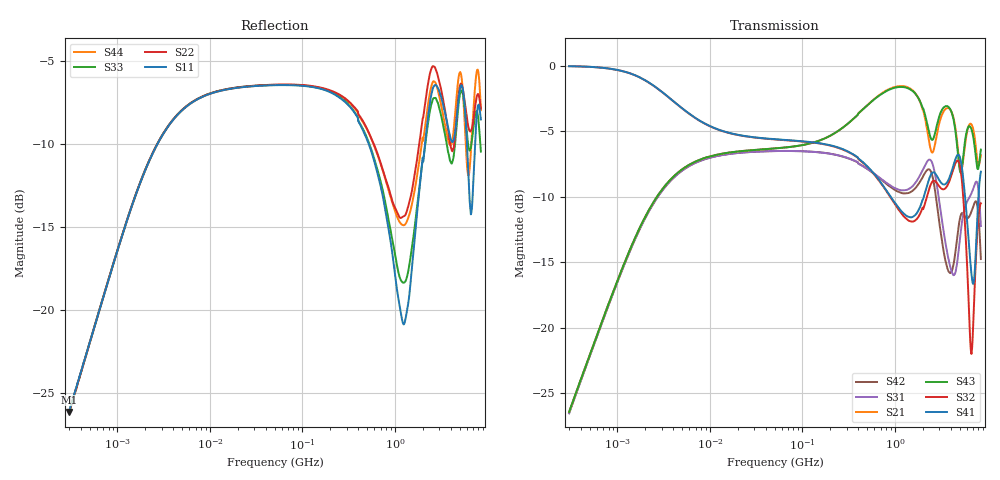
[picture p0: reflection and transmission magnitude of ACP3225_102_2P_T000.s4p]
! S-Parameter Data Generated by TDK Corporation
! Copyright(C) 2020 TDK Corporation.
! All Rights Reserved.
! TDK P/N: ACP3225-102-2P-T000 (Common Mode Filter)
! Property: |Zc|=1000ohm at 100MHz
! Size(LxWxT): 3.2x2.5x1.9mm
! Model Type: s4p (Touchstone File Format Version 1.0)
! Frequency: DC=Yes Start=0.3MHz Stop=8500MHz 802points Log-sweep
! Model Generated on Aug. 18, 2020
! Port Assignments:
!  1 ---@@@--- 4
!  2 ---@@@--- 3
! Applicable Conditions:
!  Temperature = 25 degC
!  DC Bias Current = 0 A
!  Small Signal Operation
! Terms and conditions regarding TDK Simulation Models
! (1)This simulation model is being provided solely for informational purposes. Please refer to the specifications of the products in terms of detailed characteristics of such products.
! (2)In no event shall TDK Corporation of any of its subsidiaries be liable for any loss or damage arising, directly or indirectly,
!  From any information contained in this simulation model, including, but not limited to loss or damages arising from any inaccuracies, omissions or errors in connection with such information.
! (3)Any and all copyrights on this simulation model are owned by TDK Corporation.
!  Duplication or redistribution of this simulation model without prior written permission from TDK Corporation is prohibited.
! (4)This simulation model is subject to any modification or change without any prior notice.
! (5)Neither TDK Corporation nor any of its subsidiaries shall make any warranty, express or implied,
!  Including but not limited to the correctness, implied warranties of merchantability and fitness for a particular purpose with respect to this simulation models.
! (6)The use of this simulation model shall be deemed to have consented to the terms and conditions hereof.
# Hz S MA R 50
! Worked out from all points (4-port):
!   801 points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, 300 kHz to 8.5 GHz, reference 50 ohm
!   strongest paths, dB at 300 kHz, 3.892 MHz, 50.5 MHz, 655.2 MHz, 8.5 GHz:
!     S41: 0.0, -2.6, -5.6, -8.6, -8.1
!     S32: -0.1, -2.6, -5.6, -8.7, -10.5
!     S43: -26.4, -8.6, -6.3, -2.4, -6.4
!     S21: -26.4, -8.6, -6.3, -2.3, -6.9
!     S31: -26.5, -8.7, -6.5, -8.5, -12.2
!     S42: -26.5, -8.7, -6.5, -8.5, -14.8
!   lowest |S11| = -26.1 dB at 300 kHz (marker M1), VSWR 1.10, Z = 50.2 + j4.94 ohm
!   |S11| at or under -10 dB: start of sweep to 2.704 MHz; 521 MHz to 2.114 GHz (1.593 GHz wide, 121 % of centre); 6.015 GHz to 7.348 GHz (1.333 GHz wide, 20 % of centre)
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300000  0.0493 84.9  0.04772 83.8  0.04725 -96.3  0.9957 -2.8
        0.04763 83.8  0.04881 84.0  0.9948 -2.7  0.0472 -96.3
        0.04712 -96.3  0.9942 -2.7  0.04936 84.4  0.04773 83.6
        0.9945 -2.7  0.0472 -96.3  0.04772 83.7  0.04916 84.6
8938596  0.4428 18.0  0.445 19.5  0.4401 -162.4  0.5992 -14.9
         0.445 19.5  0.4439 18.2  0.5982 -15.0  0.4401 -162.2
         0.4401 -162.4  0.5981 -15.0  0.4438 18.0  0.4451 19.5
         0.5992 -14.9  0.44 -162.2  0.4451 19.5  0.4428 18.2
1.010223e9  0.1257 -51.6  0.8295 -9.6  0.3402 75.5  0.2984 -91.3
            0.8294 -9.6  0.2024 -30.1  0.2941 -93.1  0.3344 89.8
            0.3401 75.4  0.2942 -93.1  0.1454 -47.8  0.8237 -9.6
            0.298 -91.3  0.3342 89.9  0.8238 -9.6  0.1972 -32.3
2.784768e9  0.4754 -73.5  0.526 -30.4  0.3665 -52.3  0.3842 108.6
            0.5252 -30.3  0.5265 -74.5  0.362 96.4  0.313 -50.7
            0.3653 -52.2  0.3592 96.2  0.4328 -81.3  0.5737 -33.9
            0.3833 108.7  0.3127 -50.6  0.5741 -33.9  0.4787 -73.2
5.489348e9  0.452 -99.1  0.4371 -58.1  0.2711 58.6  0.3666 -63.1
            0.4404 -57.4  0.4544 -94.1  0.3129 -84.3  0.2728 59.6
            0.2716 59.8  0.3125 -82.3  0.4391 -103.2  0.4541 -61.2
            0.3683 -63.6  0.2714 59.7  0.4525 -60.6  0.435 -96.7
6.718408e9  0.1967 -77.5  0.5953 -82.3  0.3202 -18.8  0.1609 -151.1
            0.5966 -83.0  0.3493 -87.1  0.08083 138.7  0.2786 -8.7
            0.3251 -18.1  0.07934 145.6  0.3169 -89.9  0.569 -90.9
            0.1601 -149.9  0.2769 -8.1  0.5716 -91.2  0.3187 -54.0
8.5e9  0.375 -136.8  0.4564 -99.7  0.2406 -115.5  0.3923 12.3
       0.4541 -99.3  0.404 -116.3  0.299 -8.1  0.1779 -116.4
       0.2441 -115.9  0.2982 -7.0  0.3 -126.1  0.4792 -107.5
       0.3935 12.0  0.1827 -117.4  0.4777 -107.5  0.3998 -127.9
